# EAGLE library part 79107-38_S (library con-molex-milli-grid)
RECEPTACAL
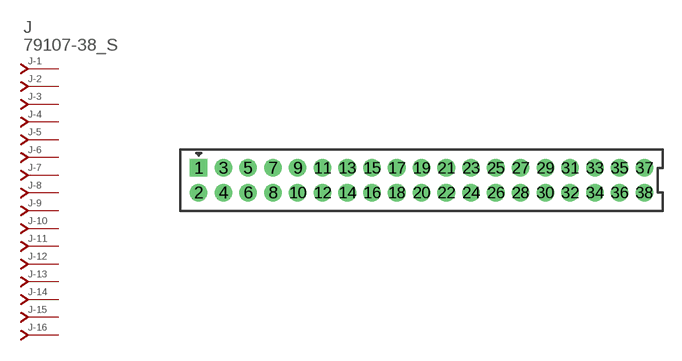
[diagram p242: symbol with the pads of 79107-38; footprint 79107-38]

Designator prefix J; gates -1=J-NV -2=J-N -3=J-N -4=J-N -5=J-N -6=J-N -7=J-N -8=J-N -9=J-N -10=J-N -11=J-N -12=J-N -13=J-N -14=J-N -15=J-N -16=J-N -17=J-N -18=J-N -19=J-N -20=J-N -21=J-N -22=J-N -23=J-N -24=J-N -25=J-N -26=J-N -27=J-N -28=J-N -29=J-N -30=J-N -31=J-N -32=J-N -33=J-N -34=J-N -35=J-N -36=J-N -37=J-N -38=J-N

## 79107-38_S  [79107-38]
1  -1:J  pas
2  -2:J  pas
3  -3:J  pas
4  -4:J  pas
5  -5:J  pas
6  -6:J  pas
7  -7:J  pas
8  -8:J  pas
9  -9:J  pas
10  -10:J  pas
11  -11:J  pas
12  -12:J  pas
13  -13:J  pas
14  -14:J  pas
15  -15:J  pas
16  -16:J  pas
17  -17:J  pas
18  -18:J  pas
19  -19:J  pas
20  -20:J  pas
21  -21:J  pas
22  -22:J  pas
23  -23:J  pas
24  -24:J  pas
25  -25:J  pas
26  -26:J  pas
27  -27:J  pas
28  -28:J  pas
29  -29:J  pas
30  -30:J  pas
31  -31:J  pas
32  -32:J  pas
33  -33:J  pas
34  -34:J  pas
35  -35:J  pas
36  -36:J  pas
37  -37:J  pas
38  -38:J  pas

## Footprint 79107-38 (pad centres in mm)
RECEPTACAL Dual Row, Vertical, Through-Hole
drill 0.914 square: 1 -18,1
drill 0.914: 2 -18,-1; 3 -16,1; 4 -16,-1; 5 -14,1; 6 -14,-1; 7 -12,1; 8 -12,-1; 9 -10,1; 10 -10,-1; 11 -8,1; 12 -8,-1; 13 -6,1; 14 -6,-1; 15 -4,1; 16 -4,-1; 17 -2,1; 18 -2,-1; 19 0,1; 20 0,-1; 21 2,1; 22 2,-1; 23 4,1; 24 4,-1; 25 6,1; 26 6,-1; 27 8,1; 28 8,-1; 29 10,1; 30 10,-1; 31 12,1; 32 12,-1; 33 14,1; 34 14,-1; 35 16,1; 36 16,-1; 37 18,1; 38 18,-1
